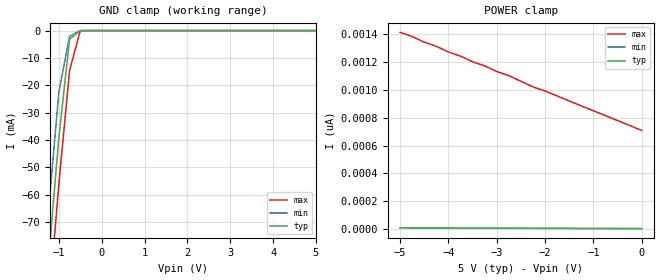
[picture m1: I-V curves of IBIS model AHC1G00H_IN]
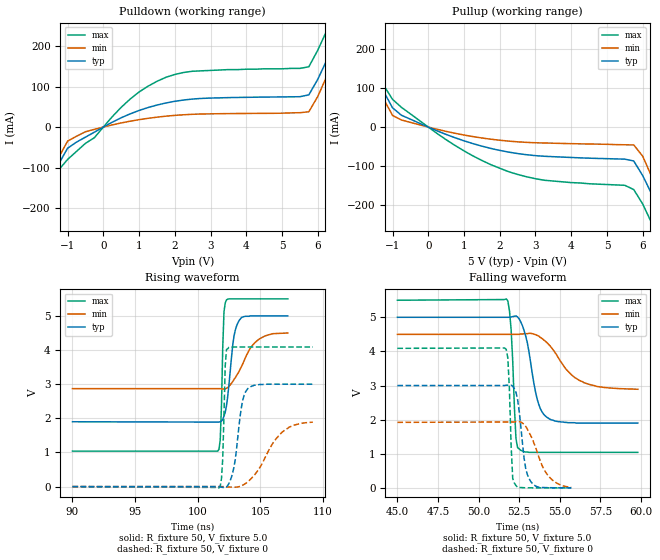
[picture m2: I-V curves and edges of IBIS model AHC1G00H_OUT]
| TEXAS INSTRUMENTS INCORPORATED
| Standard Linear and Logic Group
| IBIS Model of SN74AHC1G00H
| SINGLE 2-INPUT POSITIVE-NAND GATE
| CMPAK-5 5-pin (DCK) Package
[IBIS Ver]   2.1
[Comment Char]  |_char
[File name]   ul00_5c.ibs
[File Rev]   2.0
[Date]   April 17, 2000
[Source]   Data created from SPICE simulations at Hitachi,Ltd.
[Notes]   The following is an IBIS List for the AHC1G00H.
|   Please contact sllibis@ti.com with questions and
|   comments concerning SLL IBIS models.
[Disclaimer] Property of Texas Instruments Incorporated.  Unauthorized
   reproduction and/or distribution is strictly prohibited.
   This product is protected under copyright law.
   Created 2000, (C) Copyright 2000, Texas Instruments Inc.,
   All Rights Reserved.
   UNLESS THERE IS A SIGNED, WRITTEN AGREEMENT TO THE
   CONTRARY, TEXAS INSTRUMENTS () IS PROVIDING THE IBIS
   MODELS  AND WITHOUT ANY WARRANTY, EXPRESSED OR
   IMPLIED.  TI assumes no liability for:
   1) the accuracy of the IBIS models provided to your
   company;
   2) the proper functioning of these IBIS Models in your
   design or for any resulting applications; or
   3) infringement of patents, copyrights or intellectual
   property rights resulting from your use of these IBIS
   models.
   TI provides IBIS Models as a service to our customers.
   You and your company shall not distribute, sell or give
   these models to anyone else without prior written
   permission from TI.
   TI reserves the right to make changes to our products or
   to discontinue any semiconductor product or service
   without notice, and advises our customers to obtain the
   latest version of relevant information to verify, before
   placing orders, that the information being relied on is
   current.
   Please be aware that your receipt and use of the IBIS
   information provided shall serve as acceptance of these
   terms and conditions.  If you do not accept these terms,
   you should return or destroy the IBIS models and any
   other accompanying information immediately.
|   Component AHC1G00H
[Component]   AHC1G00H
[Manufacturer]   Hitachi, Ltd.
[Package]
|   typ   min   max
R_pkg   0.090   0.051   0.105
L_pkg   1.500nH   0.940nH   1.700nH
C_pkg   0.170pF   0.110pF   0.360pF
[Pin]   signal_name   model_name   R_pin   L_pin   C_pin
1   A   AHC1G00H_IN   0.098   1.590nH   0.110pF
2   B   AHC1G00H_IN   0.051   0.940nH   0.170pF
3   GND   GND   0.092   1.590nH   0.360pF
4   Y   AHC1G00H_OUT   0.105   1.700nH   0.110pF
5   VCC   POWER   0.104   1.690nH   0.110pF
| Models and submodels in the file (2): AHC1G00H_IN (Input), AHC1G00H_OUT (Output)
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|   Model AHC1G00H_IN
[Model]   AHC1G00H_IN
Model_type  Input
Polarity   Inverting
Vinl = 1.50
Vinh = 3.50
| variable   typ   min   max
C_comp   2.19pF   2.07pF   2.30pF
[Temperature Range]   25   85   -40
[Voltage Range]   5.0   4.5   5.5
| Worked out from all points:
|   GND clamp passes 1 mA (typ) near -0.58 V on its own axis
[GND Clamp]
|   Voltage   I(typ)   I(min)   I(max)
-5V       -823mA     -807mA     -840mA
-1.5V     -133mA     -115mA     -150mA
-1.25V    -85.2mA    -67.5mA    -103mA
-1V       -39.2mA    -22.5mA    -56.2mA
-750mV    -3.18mA    -2.09mA    -14.6mA
-500mV    -11.6uA    -2.99uA    -57.1uA
5V        5.34pA     5pA        708pA
[POWER Clamp]
|   Voltage   I(typ)   I(min)   I(max)
-5V       10.6pA     10pA       1.41nA
-4.75V    10.3pA     9.75pA     1.38nA
-4.5V     10pA       9.5pA      1.34nA
-4.25V    9.78pA     9.25pA     1.31nA
-4V       9.52pA     9pA        1.27nA
-3.75V    9.26pA     8.75pA     1.24nA
-3.5V     9pA        8.5pA      1.2nA
-3.25V    8.74pA     8.25pA     1.17nA
-2.75V    8.21pA     7.75pA     1.1nA
-2.25V    7.69pA     7.25pA     1.02nA
-2V       7.43pA     7pA        990pA
0V        5.34pA     5pA        708pA
|   Model AHC1G00H_OUT
[Model]   AHC1G00H_OUT
Model_type  Output
Polarity   Non-Inverting
Vmeas = 2.5
Cref = 15pf
| variable   typ   min   max
C_comp   4.52pF   4.32pF   4.72pF
[Temperature Range]   25   85   -40
[Voltage Range]   5.0   4.5   5.5
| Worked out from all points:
|   slope of the pulldown table from 0 to 0.75 V, typ, clamps not added: 23 ohm
|   slope of the pullup table from 0 to 0.75 V, typ, clamps not added: 27.3 ohm
|   rising waveform, R_fixture 50, V_fixture 5.0: 20-80 % time 535ps typ, 1.45ns min, 196ps max; typ from 1.9 V to 5 V
|   falling waveform, R_fixture 50, V_fixture 5.0: 20-80 % time 721ps typ, 1.63ns min, 244ps max; typ from 5 V to 1.9 V
|   falling waveform, R_fixture 50, V_fixture 0: 20-80 % time 435ps typ, 1.02ns min, 189ps max; typ from 3 V to 0.001 V
|   rising waveform, R_fixture 50, V_fixture 0: 20-80 % time 621ps typ, 1.92ns min, 183ps max; typ from 0 V to 3 V
[Pulldown]
|   Voltage   I(typ)   I(min)   I(max)
-5V       -826mA     -810mA     -842mA
-2.25V    -282mA     -267mA     -299mA
-2V       -234mA     -219mA     -250mA
-1.25V    -91.3mA    -75.2mA    -106mA
-1V       -52.3mA    -34.7mA    -80mA
750mV     32.6mA     14.5mA     69.2mA
1.75V     59.5mA     26.9mA     123mA
5.75V     79.6mA     37.8mA     149mA
6.25V     165mA      125mA      238mA
6.75V     261mA      217mA      336mA
7V        310mA      265mA      385mA
10V       906mA      861mA      980mA
[Pullup]
|   Voltage   I(typ)   I(min)   I(max)
-5V       828mA      811mA      845mA
-2.25V    284mA      267mA      301mA
-2V       235mA      218mA      252mA
-1V       49.6mA     30.1mA     71.4mA
750mV     -27.5mA    -16mA      -47.4mA
2.25V     -64.5mA    -36.2mA    -115mA
5.75V     -87.4mA    -46mA      -161mA
6V        -125mA     -75mA      -198mA
6.25V     -172mA     -127mA     -247mA
6.75V     -269mA     -224mA     -345mA
7V        -318mA     -273mA     -395mA
10V       -917mA     -874mA     -991mA
[Ramp]
| variable   typ   min   max
dV/dt_r   1.80E+00/6.10E-10   1.14E+00/1.94E-09   2.45E+00/1.80E-10
dV/dt_f   1.86E+00/7.20E-10   9.76E-01/1.68E-09   2.68E+00/2.40E-10
R_load = 50
[Rising Waveform]
R_fixture = 50
V_fixture = 5.0
V_fixture_min = 4.5
V_fixture_max = 5.5
|   Time   V(typ)   V(min)   V(max)
90ns      1.9V       2.87V      1.04V
101.6ns   1.89V      2.87V      1.04V
101.8ns   1.9V       2.87V      1.37V
101.9ns   1.92V      2.86V      2.39V
102.1ns   2.06V      2.86V      5.12V
102.3ns   2.37V      2.88V      5.47V
102.9ns   4.41V      3.14V      5.5V
103.3ns   4.86V      3.37V      5.5V
104.9ns   5V         4.32V      5.5V
107.2ns   5V         4.5V       5.5V
[Falling Waveform]
R_fixture = 50
V_fixture = 5.0
V_fixture_min = 4.5
V_fixture_max = 5.5
|   Time   V(typ)   V(min)   V(max)
45ns      5V         4.5V       5.5V
51.7ns    5V         4.5V       5.54V
52ns      5.01V      4.5V       4.65V
52.3ns    5.04V      4.5V       1.44V
52.6ns    4.86V      4.51V      1.1V
53ns      4.25V      4.52V      1.05V
53.6ns    2.61V      4.47V      1.04V
54.1ns    2.11V      4.3V       1.04V
56.2ns    1.9V       3.15V      1.04V
59.8ns    1.9V       2.89V      1.04V
[Falling Waveform]
R_fixture = 50
V_fixture = 0
|   Time   V(typ)   V(min)   V(max)
45ns      3V         1.92V      4.09V
51.6ns    3V         1.93V      4.1V
51.8ns    3.01V      1.93V      3.8V
52.1ns    2.98V      1.93V      274mV
52.2ns    2.91V      1.93V      138mV
52.4ns    2.59V      1.94V      14.1mV
52.9ns    567mV      1.8V       2.25mV
53.2ns    193mV      1.54V      462uV
54.3ns    5.3mV      346mV      33uV
55.7ns    507uV      14.7mV     11uV
[Rising Waveform]
R_fixture = 50
V_fixture = 0
|   Time   V(typ)   V(min)   V(max)
90ns      0V         0V         0V
101.7ns   -2.2mV     416uV      -36.5mV
102ns     -23mV      85uV       826mV
102.2ns   -27mV      -4.97mV    3.54V
102.3ns   -9.7mV     -8.13mV    4.02V
102.9ns   577mV      -16.8mV    4.09V
103.5ns   2.34V      24.9mV     4.09V
104ns     2.87V      142mV      4.09V
106.7ns   3V         1.58V      4.09V
109.2ns   3V         1.89V      4.09V
